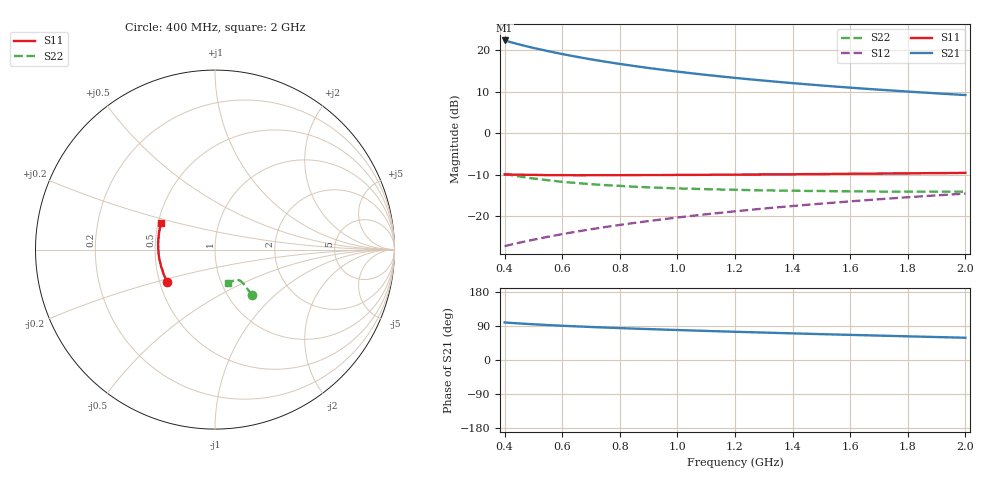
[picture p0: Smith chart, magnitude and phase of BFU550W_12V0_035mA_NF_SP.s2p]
! Filename:  P:\Prog\Test\Noise\ATS_data\Testdata_Net\06 Compressed Noise after Statistics\BFU550W_APM2013_11_D05_12p0V_035mA_NF_CM01_D.sf
! Date/Time: Tue 26/Mar/2013 16:25:27
! BFU550W_APM2013_11_D05_12p0V_1to35mA_NF_CM01_Bias9_R.sf
! Noise Parameter Data File
! BFU550W_APM2013_11_D05_12p0V_1to35mA_NF_CM01
! Date/time: Mon Mar 25 15:58:35 2013
! VAR V_out= 12.001000
! VAR I_out= 34.990000
! VAR V_in= 0.723200
! VAR I_in= 0.319700
! Device data file deembeded for feedlines and parallel
! Original file: \06 Compressed Noise after Statistics\BFU550W_APM2013_11_D05_12p0V_035mA_NF_CM01_R.sf
! Feed-files: PR019V01_070313_Feed1.s2p, PR019V01_070313_Feed2.s2p
! Parallel-file: PR019V01_070313_Par.s2p
# MHz S MA R 50
!  Freq-MHz  S11-mag  S11-arg  S21-mag  S21-arg  S12-mag  S12-arg  S22-mag  S22-arg
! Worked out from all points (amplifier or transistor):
!   37 points, 400 MHz to 2 GHz, reference 50 ohm
!   highest |S21| = 22.4 dB at 400 MHz (marker M1)
!   |S21| within 3 dB of that: start of sweep to 581.1 MHz
!   unconditionally stable (mu >= 1): 959.5 MHz to end of sweep
!   at 500 MHz: K = 0.93, MSG = 23.1 dB, |S12| = -25.6 dB
!   at 1.1 GHz: K = 1.01, MAG = 16.3 dB, |S12| = -19.5 dB
!   at 2 GHz: K = 1.00, MAG = 11.5 dB, |S12| = -14.5 dB
!   lowest NFmin = 1.33 dB at 400 MHz
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400  0.3202 -145.9  13.14 99.0  0.0439 68.8  0.3253 -50.7
420  0.3195 -148.0  12.57 98.0  0.04565 69.1  0.3164 -50.7
440  0.3187 -150.0  12.04 97.0  0.04736 69.4  0.3077 -50.6
460  0.3179 -151.8  11.55 96.1  0.04908 69.7  0.3001 -50.6
480  0.3172 -153.6  11.11 95.2  0.0508 69.9  0.2933 -50.6
500  0.3171 -155.4  10.69 94.3  0.0525 70.1  0.2866 -50.5
550  0.3143 -159.0  9.791 92.2  0.05691 70.7  0.2729 -50.4
600  0.3147 -162.3  9.02 90.4  0.06129 71.0  0.2612 -50.2
650  0.3135 -165.2  8.359 88.7  0.06575 71.3  0.2526 -50.2
700  0.314 -168.0  7.788 87.1  0.07019 71.5  0.2449 -50.3
750  0.3145 -170.3  7.295 85.7  0.07464 71.7  0.2384 -50.3
800  0.3141 -172.8  6.858 84.2  0.07914 71.8  0.2334 -50.7
850  0.3151 -175.0  6.472 82.8  0.08355 71.8  0.2282 -50.7
950  0.3152 -178.8  5.82 80.3  0.09264 71.8  0.2209 -51.4
1050  0.3165 177.8  5.29 77.9  0.1017 71.6  0.2155 -52.3
1150  0.3188 174.3  4.849 75.6  0.1107 71.3  0.2112 -53.4
1200  0.3187 173.0  4.66 74.5  0.1154 71.1  0.2095 -54.1
1350  0.3213 168.7  4.168 71.3  0.1291 70.5  0.2049 -56.0
1500  0.324 164.8  3.775 68.2  0.1428 69.6  0.2027 -58.5
1650  0.3273 161.0  3.453 65.3  0.1565 68.7  0.2005 -61.0
1750  0.3294 158.9  3.273 63.4  0.1657 68.1  0.1992 -62.9
2000  0.3351 153.3  2.896 58.7  0.1885 66.3  0.1984 -68.3
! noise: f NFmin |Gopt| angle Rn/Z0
400  1.335  0.3212  -173.4  0.0873
460  1.337  0.3203  -171.8  0.0905
600  1.367  0.3341  -166.8  0.0886
800  1.403  0.3348  -164.4  0.0903
1000  1.427  0.3444  -160.2  0.093
1200  1.459  0.3482  -156.4  0.0997
1400  1.486  0.3572  -152.7  0.1048
1600  1.519  0.3685  -148.1  0.1096
1800  1.582  0.3804  -143.3  0.1144
2000  1.571  0.3949  -140.9  0.1236
